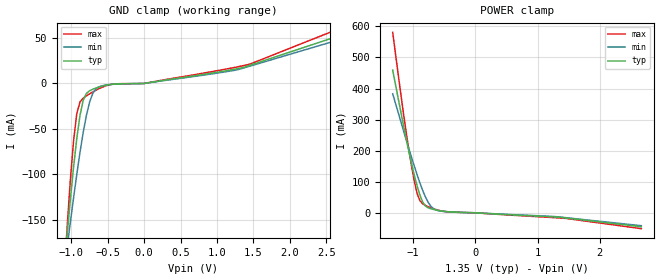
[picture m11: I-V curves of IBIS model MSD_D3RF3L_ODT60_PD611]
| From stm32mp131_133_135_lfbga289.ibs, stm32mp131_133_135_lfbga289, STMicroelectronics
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[Model] MSD_D3RF3L_ODT60_PD611
Model_type   Input
C_comp 2.393pF   2.343pF   2.462pF
Vinh = 810.000mV
Vinl = 540.000mV
[Receiver Thresholds]
Vth   =  0.675V
Vth_min  =  0.6615V
Vth_max  =  0.6885V
Vinh_ac  =  0.160V
Vinh_dc  =  0.090V
Vinl_ac  = -0.160V
Vinl_dc  = -0.090V
Tslew_ac =  5.000ns |Not specified, so set to high value
[Temperature Range]   25.000   125.000   -40.000
[Voltage Range]   1.350V   1.283V   1.450V
[GND Clamp Reference]   0.00V   0.00V   0.00V
[POWER Clamp Reference]   1.350V   1.283V   1.450V
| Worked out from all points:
|   GND clamp passes 1 mA (typ) near -0.45 V on its own axis
|   POWER clamp passes 1 mA (typ) near -0.18 V on its own axis
[GND Clamp]
-1.318V   -430mA     -356.9mA   -545.3mA
-1.098V   -209.2mA   -209.7mA   -216.9mA
-1.055V   -167.7mA   -181.2mA   -158.9mA
-1.011V   -128.5mA   -153.3mA   -106.9mA
-966.7mV  -92.45mA   -126.3mA   -63.5mA
-922.7mV  -60.77mA   -100.4mA   -33.42mA
-834.9mV  -18.73mA   -54.15mA   -16.16mA
-747mV    -8.026mA   -20.62mA   -11.43mA
-659.1mV  -5.022mA   -5.89mA    -7.41mA
-571.2mV  -2.849mA   -2.478mA   -4.028mA
1.45V     19.96mA    19.07mA    21.27mA
2.68V     52.67mA    48.37mA    60.53mA
[Power Clamp]
-1.33V    459.1mA    383.1mA    580.7mA
-1.155V   279.5mA    263.1mA    316.6mA
-1.023V   154.8mA    175.8mA    145.5mA
-978.8mV  118mA      147.7mA    97.92mA
-934.9mV  84.64mA    120.7mA    60.52mA
-890.9mV  55.88mA    95.1mA     38.5mA
-847mV    34.14mA    71.48mA    28.65mA
-803mV    21.61mA    50.61mA    23.52mA
-715.1mV  12.86mA    20.63mA    16.01mA
-583.3mV  6.938mA    6.198mA    7.68mA
1.438V    -16.29mA   -15.46mA   -17.88mA
2.668V    -44.94mA   -41.61mA   -51.13mA
